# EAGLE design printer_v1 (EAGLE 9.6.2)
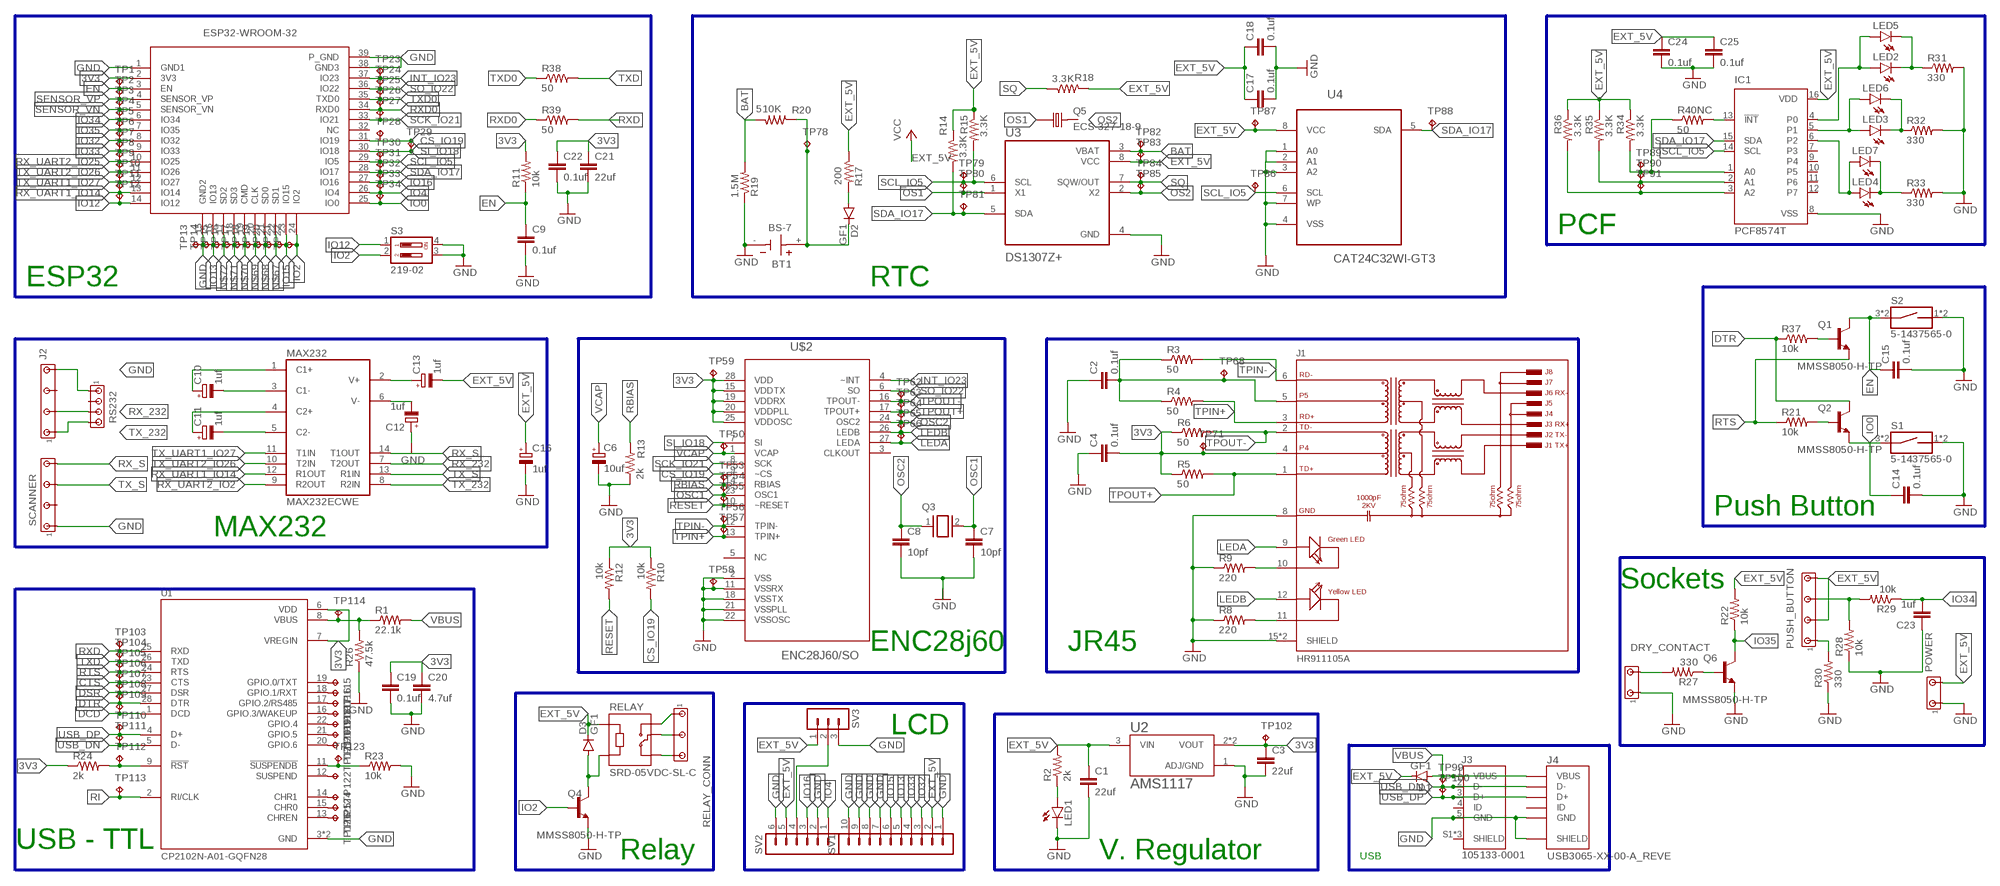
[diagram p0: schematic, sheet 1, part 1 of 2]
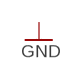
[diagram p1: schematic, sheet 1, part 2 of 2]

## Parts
BT1  BS-7  [BAT_BS-7]
C1  22uf  C-EUC1206  [C1206]
C2  0.1uf  C-EUC1206  [C1206]
C3  22uf  C-EUC1206  [C1206]
C4  0.1uf  C-EUC1206  [C1206]
C6  10uf  CPOL-EU153CLV-0405  [153CLV-0405]
C7  10pf  C-EUC1206  [C1206]
C8  10pf  C-EUC1206  [C1206]
C9  0.1uf  C-EUC1206  [C1206]
C10  1uf  CPOL-EU153CLV-0405  [153CLV-0405]
C11  1uf  CPOL-EU153CLV-0405  [153CLV-0405]
C12  1uf  CPOL-EU153CLV-0405  [153CLV-0405]
C13  1uf  CPOL-EU153CLV-0405  [153CLV-0405]
C14  0.1uf  C-EUC1206  [C1206]
C15  0.1uf  C-EUC1206  [C1206]
C16  1uf  CPOL-EU153CLV-0405  [153CLV-0405]
C17  0.1uf  C-EUC1206  [C1206]
C18  0.1uf  C-EUC1206  [C1206]
C19  0.1uf  C-EUC1206  [C1206]
C20  4.7uf  C-EUC1206  [C1206]
C21  22uf  C-EUC1206  [C1206]
C22  0.1uf  C-EUC1206  [C1206]
C23  1uf  C-EUC1206  [C1206]
C24  0.1uf  C-EUC1206  [C1206]
C25  0.1uf  C-EUC1206  [C1206]
D1  GF1  [SMA-DO214AC]
D2  GF1  [SMA-DO214AC]
D3  GF1  [SMA-DO214AC]
DRY_CONTACT  MTA03-100_MYV  [10X03MTA_MYV]
IC1  PCF8574T  [SO16W]
J1  HR911105A  [HANRUN_HR911105A]
J2  MTA07-100_MYV  [10X07MTA_MYV]
J3  105133-0001  [MOLEX_105133-0001]
J4  USB3065-XX-00-A_REVE  [GCT_USB3065-XX-00-A_REVE]
LED1  LEDSML0603  [SML0603]
LED2  LEDSML0603  [SML0603]
LED3  LEDSML0603  [SML0603]
LED4  LEDSML0603  [SML0603]
LED5  LED5MM  [LED5MM]
LED6  LED5MM  [LED5MM]
LED7  LED5MM  [LED5MM]
MAX232  MAX232ECWE  [SO16L]
POWER  MTA03-100_MYV  [10X03MTA_MYV]
PUSH_BUTTON  MTA07-100_MYV  [10X07MTA_MYV]
Q1  MMSS8050-H-TP  [TRANS_MMSS8050-H-TP]
Q2  MMSS8050-H-TP  [TRANS_MMSS8050-H-TP]
Q3  XTAL/S  [QS]
Q4  MMSS8050-H-TP  [TRANS_MMSS8050-H-TP]
Q5  ECS-327-18-9  [XTAL_ECS-160-18-9X]
Q6  MMSS8050-H-TP  [TRANS_MMSS8050-H-TP]
R1  22.1k  R-US_R1206  [R1206]
R2  2k  R-US_R1206  [R1206]
R3  50  R-US_R1206  [R1206]
R4  50  R-US_R1206  [R1206]
R5  50  R-US_R1206  [R1206]
R6  50  R-US_R1206  [R1206]
R8  220  R-US_R1206  [R1206]
R9  220  R-US_R1206  [R1206]
R10  10k  R-US_R0805  [R0805]
R11  10k  R-US_R0805  [R0805]
R12  10k  R-US_R0805  [R0805]
R13  2k  R-US_R1206  [R1206]
R14  3.3K  R-US_R1206  [R1206]
R15  3.3K  R-US_R1206  [R1206]
R17  200  R-US_R1206  [R1206]
R18  3.3K  R-US_R1206  [R1206]
R19  1.5M  R-US_R1206  [R1206]
R20  510K  R-US_R1206  [R1206]
R21  10k  R-US_R0805  [R0805]
R22  10k  R-US_R0805  [R0805]
R23  10k  R-US_R0805  [R0805]
R24  2k  R-US_R1206  [R1206]
R26  47.5k  R-US_R1206  [R1206]
R27  330  R-US_R0402  [R0402]
R28  10k  R-US_R0805  [R0805]
R29  10k  R-US_R0805  [R0805]
R30  330  R-US_R1206  [R1206]
R31  330  R-US_R1206  [R1206]
R32  330  R-US_R1206  [R1206]
R33  330  R-US_R1206  [R1206]
R34  3.3K  R-US_R1206  [R1206]
R35  3.3K  R-US_R1206  [R1206]
R36  3.3K  R-US_R1206  [R1206]
R37  10k  R-US_R0805  [R0805]
R38  50  R-US_R0402  [R0402]
R39  50  R-US_R0402  [R0402]
R40NC  50  R-US_R0402  [R0402]
RELAY  SRD-05VDC-SL-C  [RELAY_SRD-05VDC-SL-C]
RELAY_CONN  MTA05-156_MYVSPACE1  [10X05MTA_MYV]
RS232  MTA04-100  [10X04MTA]
S1  5-1437565-0  [SW_5-1437565-0]
S2  5-1437565-0  [SW_5-1437565-0]
S3  219-02  [CTS-219-02]
SCANNER  MTA07-100_MYV  [10X07MTA_MYV]
SV1  MA10-1  [MA10-1]
SV2  MA06-1  [MA06-1]
SV3  MA03-1  [MA03-1]
TP1  TPTP06R  [TP06R]
TP2  TPTP06R  [TP06R]
TP3  TPTP06R  [TP06R]
TP4  TPTP06R  [TP06R]
TP5  TPTP06R  [TP06R]
TP6  TPTP06R  [TP06R]
TP7  TPTP06R  [TP06R]
TP8  TPTP06R  [TP06R]
TP9  TPTP06R  [TP06R]
TP10  TPTP06R  [TP06R]
TP11  TPTP06R  [TP06R]
TP12  TPTP06R  [TP06R]
TP13  TPTP06R  [TP06R]
TP14  TPTP06R  [TP06R]
TP15  TPTP06R  [TP06R]
TP16  TPTP06R  [TP06R]
TP17  TPTP06R  [TP06R]
TP18  TPTP06R  [TP06R]
TP19  TPTP06R  [TP06R]
TP20  TPTP06R  [TP06R]
TP21  TPTP06R  [TP06R]
TP22  TPTP06R  [TP06R]
TP23  TPTP06R  [TP06R]
TP24  TPTP06R  [TP06R]
TP25  TPTP06R  [TP06R]
TP26  TPTP06R  [TP06R]
TP27  TPTP06R  [TP06R]
TP28  TPTP06R  [TP06R]
TP29  TPTP06R  [TP06R]
TP30  TPTP06R  [TP06R]
TP31  TPTP06R  [TP06R]
TP32  TPTP06R  [TP06R]
TP33  TPTP06R  [TP06R]
TP34  TPTP06R  [TP06R]
TP50  TPTP06R  [TP06R]
TP53  TPTP06R  [TP06R]
TP54  TPTP06R  [TP06R]
TP55  TPTP06R  [TP06R]
TP56  TPTP06R  [TP06R]
TP57  TPTP06R  [TP06R]
TP58  TPTP06R  [TP06R]
TP59  TPTP06R  [TP06R]
TP62  TPTP06R  [TP06R]
TP63  TPTP06R  [TP06R]
TP64  TPTP06R  [TP06R]
TP65  TPTP06R  [TP06R]
TP66  TPTP06R  [TP06R]
TP68  TPTP06R  [TP06R]
TP71  TPTP06R  [TP06R]
TP78  TPTP06R  [TP06R]
TP79  TPTP06R  [TP06R]
TP80  TPTP06R  [TP06R]
TP81  TPTP06R  [TP06R]
TP82  TPTP06R  [TP06R]
TP83  TPTP06R  [TP06R]
TP84  TPTP06R  [TP06R]
TP85  TPTP06R  [TP06R]
TP86  TPTP06R  [TP06R]
TP87  TPTP06R  [TP06R]
TP88  TPTP06R  [TP06R]
TP89  TPTP06R  [TP06R]
TP90  TPTP06R  [TP06R]
TP91  TPTP06R  [TP06R]
TP99  TPTP06R  [TP06R]
TP100  TPTP06R  [TP06R]
TP102  TPTP06R  [TP06R]
TP103  TPTP06R  [TP06R]
TP104  TPTP06R  [TP06R]
TP105  TPTP06R  [TP06R]
TP106  TPTP06R  [TP06R]
TP107  TPTP06R  [TP06R]
TP108  TPTP06R  [TP06R]
TP109  TPTP06R  [TP06R]
TP110  TPTP06R  [TP06R]
TP111  TPTP06R  [TP06R]
TP112  TPTP06R  [TP06R]
TP113  TPTP06R  [TP06R]
TP114  TPTP06R  [TP06R]
TP115  TPTP06R  [TP06R]
TP116  TPTP06R  [TP06R]
TP117  TPTP06R  [TP06R]
TP118  TPTP06R  [TP06R]
TP119  TPTP06R  [TP06R]
TP120  TPTP06R  [TP06R]
TP121  TPTP06R  [TP06R]
TP122  TPTP06R  [TP06R]
TP123  TPTP06R  [TP06R]
TP124  TPTP06R  [TP06R]
TP125  TPTP06R  [TP06R]
TP126  TPTP06R  [TP06R]
U1  CP2102N-A01-GQFN28  [QFN50P500X500X80-29N]
U2  AMS1117  [SOT229P700X180-4N]
U3  DS1307Z+  [SOIC127P600X175-8N]
U4  CAT24C32WI-GT3  [SOIC127P600X175-8N]
U$2  ENC28J60/SO  [SOIC127P1034X264-28N]
U$3  ESP32-WROOM-32  [ESP32-WROOM-32]

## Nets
3V3: C3.1 C4.2 C19.1 C20.1 C21.1 C22.1 J1.4 R5.1 R6.1 R10.1 R11.2 R12.1 R24.1 TP59.TP TP71.TP TP102.TP U1.6(VDD) U1.7(VREGIN) U2.2(VOUT) U2.4(VOUT) U$2.15(VDDTX) U$2.19(VDDRX) U$2.20(VDDPLL) U$2.25(VDDOSC) U$2.28(VDD) U$3.2(3V3)
BAT: R19.2 R20.2 TP82.TP U3.3(VBAT)
CS_IO19: R10.2 TP28.TP U$2.9(~CS) U$3.31(IO19)
CTS: TP106.TP U1.23(CTS)
DCD: TP109.TP U1.1(DCD)
DSR: TP107.TP U1.27(DSR)
DTR: Q2.3(C) R37.1 TP108.TP U1.28(DTR)
EN: C9.1 C15.1 Q1.3(C) R11.1 S2.3 S2.4 TP1.TP U$3.3(EN)
EXT_5V: C1.1 C13.- C16.+ C17.1 C18.1 C24.1 C25.1 D1.K(C) D3.K(C) IC1.16(VDD) POWER.3 PUSH_BUTTON.3 PUSH_BUTTON.7 R2.2 R14.1 R15.1 R17.1 R18.2 R22.2 R34.1 R35.1 R36.1 RELAY.A1 SV1.2 SV2.5 SV3.1 TP83.TP TP87.TP U2.3(VIN) U3.8(VCC) U4.8(VCC) ; supply symbol labelled VCC
GND: BT1.- C1.2 C2.1 C3.2 C4.1 C6.- C7.2 C8.2 C9.2 C12.+ C14.2 C15.2 C16.- C17.2 C18.2 C19.2 C20.2 C21.2 C22.2 C23.1 C24.2 C25.2 DRY_CONTACT.1 IC1.8(VSS) J1.8(GND) J1.15(SHIELD) J1.16(SHIELD) J2.7 J3.5(GND) J4.5(GND) J4.6(SHIELD) J4.7(SHIELD) J4.8(SHIELD) J4.9(SHIELD) LED1.C POWER.1 Q4.2(E) Q6.2(E) R8.1 R9.1 R13.1 R19.1 R23.2 R26.1 R28.1 R30.1 R31.2 R32.2 R33.2 RS232.1 S1.1 S1.2 S2.1 S2.2 S3.3 S3.4 SCANNER.1 SV1.1 SV1.7 SV1.8 SV1.9 SV1.10 SV2.2 SV2.6 SV3.3 TP13.TP TP58.TP U1.3(GND) U1.29(GND) U2.1(ADJ/GND) U3.4(GND) U4.1(A0) U4.2(A1) U4.3(A2) U4.4(VSS) U4.7(WP) U$2.2(VSS) U$2.11(VSSRX) U$2.18(VSSTX) U$2.21(VSSPLL) U$2.22(VSSOSC) U$3.1(GND1) U$3.15(GND2) U$3.38(GND3) U$3.39(P_GND)
INT_IO23: TP23.TP U$2.4(~INT) U$3.37(IO23)
IO0: C14.1 Q2.2(E) S1.3 S1.4 TP34.TP U$3.25(IO0)
IO2: Q4.1(B) S3.2 TP22.TP U$3.24(IO2)
IO4: SV2.1 TP33.TP U$3.26(IO4)
IO12: S3.1 TP12.TP U$3.14(IO12)
IO13: SV1.5 TP14.TP U$3.16(IO13)
IO15: SV1.6 TP21.TP U$3.23(IO15)
IO16: SV2.3 TP32.TP U$3.27(IO16)
IO32: SV1.3 TP6.TP U$3.8(IO32)
IO33: SV1.4 TP7.TP U$3.9(IO33)
IO34: C23.2 R29.1 TP4.TP U$3.6(IO34)
IO35: Q6.3(C) R22.1 TP5.TP U$3.7(IO35)
LEDA: J1.9(GA) TP66.TP U$2.27(LEDA)
LEDB: J1.12(YA) TP65.TP U$2.26(LEDB)
N$1: LED1.A R2.1
N$2: Q1.1(B) R37.2
N$3: Q2.1(B) R21.2
N$4: R1.1 R26.2 TP114.TP U1.8(VBUS)
N$5: SV2.4 SV3.2
N$6: R23.1 TP123.TP U1.11(!SUSPENDB)
N$7: J1.11(YC) R8.2
N$8: C2.2 J1.5 R3.1 R4.1 TP68.TP
N$9: J1.10(GC) R9.2
N$10: TP115.TP U1.19(GPIO.0/TXT)
N$11: TP116.TP U1.18(GPIO.1/RXT)
N$12: C10.+ MAX232.1(C1+)
N$13: TP117.TP U1.17(GPIO.2/RS485)
N$14: C10.- MAX232.3(C1-)
N$15: C11.- MAX232.5(C2-)
N$16: R24.2 TP112.TP U1.9(!RST)
N$17: TP118.TP U1.16(GPIO.3/WAKEUP)
N$18: C11.+ MAX232.4(C2+)
N$19: C12.- MAX232.6(V-)
N$20: C13.+ MAX232.2(V+)
N$21: RELAY.NC RELAY_CONN.5
N$22: RELAY.COM RELAY_CONN.3
N$23: LED2.C LED5.K(C) R31.1
N$24: IC1.13(!INT) R40NC.2
N$25: TP119.TP U1.22(GPIO.4)
N$26: RELAY.NO RELAY_CONN.1
N$27: D3.A Q4.3(C) RELAY.A2
N$28: D2.A R17.2
N$29: BT1.+ D2.K(C) R20.1 TP78.TP
N$30: TP120.TP U1.21(GPIO.5)
N$31: TP121.TP U1.20(GPIO.6)
N$32: Q6.1(B) R27.1
N$33: PUSH_BUTTON.5 R28.2 R29.2
N$34: TP122.TP U1.12(SUSPEND)
N$35: DRY_CONTACT.3 R27.2
N$36: IC1.4(P0) LED2.A LED5.A
N$37: IC1.5(P1) LED3.A LED6.A
N$38: IC1.6(P2) LED4.A LED7.A
N$39: TP124.TP U1.14(CHR1)
N$40: PUSH_BUTTON.1 R30.2
N$41: TP125.TP U1.15(CHR0)
N$42: TP126.TP U1.13(CHREN)
N$45: IC1.1(A0) R34.2 R40NC.1 TP89.TP
N$46: IC1.2(A1) R35.2 TP90.TP
N$47: IC1.3(A2) R36.2 TP91.TP
N$48: LED3.C LED6.K(C) R32.1
N$49: LED4.C LED7.K(C) R33.1
N$67: TP20.TP U$3.22(SD1)
N$68: TP19.TP U$3.21(SD0)
N$69: TP18.TP U$3.20(CLK)
N$70: TP17.TP U$3.19(CMD)
N$71: TP16.TP U$3.18(SD3)
N$72: TP15.TP U$3.17(SD2)
OS1: Q5.1 TP80.TP U3.1(X1)
OS2: Q5.2 TP85.TP U3.2(X2)
OSC1: C7.1 Q3.2 TP54.TP U$2.23(OSC1)
OSC2: C8.1 Q3.1 TP64.TP U$2.24(OSC2)
RBIAS: R13.2 TP53.TP U$2.14(RBIAS)
RESET: R12.2 TP55.TP U$2.10(~RESET)
RI: TP113.TP U1.2(RI/CLK)
RTS: Q1.2(E) R21.1 TP105.TP U1.24(RTS)
RX_232: J2.3 MAX232.7(T2OUT) RS232.3
RX_S: MAX232.14(T1OUT) SCANNER.7
RX_UART1_IO14: MAX232.12(R1OUT) TP11.TP U$3.13(IO14)
RX_UART2_IO2: MAX232.9(R2OUT)
RX_UART2_IO25: TP8.TP U$3.10(IO25)
RXD: R39.2 TP103.TP U1.25(RXD)
RXD0: R39.1 TP26.TP U$3.34(RXD0)
SCK_IO21: TP27.TP U$2.8(SCK) U$3.33(IO21)
SCL_IO5: IC1.14(SCL) R15.2 TP30.TP TP79.TP TP86.TP U3.6(SCL) U4.6(SCL) U$3.29(IO5)
SDA_IO17: IC1.15(SDA) R14.2 TP31.TP TP81.TP TP88.TP U3.5(SDA) U4.5(SDA) U$3.28(IO17)
SENSOR_VN: TP3.TP U$3.5(SENSOR_VN)
SENSOR_VP: TP2.TP U$3.4(SENSOR_VP)
SI_IO18: TP29.TP U$2.7(SI) U$3.30(IO18)
SO_IO22: TP24.TP U$2.6(SO) U$3.36(IO22)
SQ: R18.1 TP84.TP U3.7(SQW/OUT)
TPIN+: J1.3(RD+) R4.2 TP57.TP U$2.13(TPIN+)
TPIN-: J1.6(RD-) R3.2 TP56.TP U$2.12(TPIN-)
TPOUT+: J1.1(TD+) R5.2 TP63.TP U$2.17(TPOUT+)
TPOUT-: J1.2(TD-) R6.2 TP62.TP U$2.16(TPOUT-)
TX_232: J2.1 MAX232.8(R2IN) RS232.4
TX_S: MAX232.13(R1IN) SCANNER.5
TX_UART1_IO27: MAX232.11(T1IN) TP10.TP U$3.12(IO27)
TX_UART2_IO26: MAX232.10(T2IN) TP9.TP U$3.11(IO26)
TXD: R38.2 TP104.TP U1.26(TXD)
TXD0: R38.1 TP25.TP U$3.35(TXD0)
USB_DN: J3.2(D-) J4.2(D-) TP99.TP TP111.TP U1.5(D-)
USB_DP: J3.3(D+) J4.3(D+) TP100.TP TP110.TP U1.4(D+)
VBUS: D1.A J3.1(VBUS) J4.1(VBUS) R1.2
VCAP: C6.+ TP50.TP U$2.1(VCAP)
Unconnected: IC1.7(P3) IC1.9(P4) IC1.10(P5) IC1.11(P6) IC1.12(P7) J2.5 J3.4(ID) J3.S1(SHIELD) J3.S2(SHIELD) J3.S3(SHIELD) J4.4(ID) RS232.2 SCANNER.3 U$2.3(CLKOUT) U$2.5(NC) U$3.32(NC)

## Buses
B$1
B$2
BAT,EXT_5V,GND,N$28,N$29
B$3
B$4
B$5
B$6
B$7
GND,EXT_5V_PIN
B$8
VBUS,GND,USB_DN,N$6,3V3,RI,RTS,RXD,TXD,CTS,DSR,N$4,DTR,DCD,USB_DP,N$16
B$9
B$10

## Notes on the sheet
- PCF
- ESP32 | RTC
- Push Button
- MAX232
- Sockets
- ENC28j60 | JR45
- LCD
- USB - TTL
- Relay | V. Regulator | USB

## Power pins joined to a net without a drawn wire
EXT_5V: MAX232.16(VCC)
GND: MAX232.15(GND)

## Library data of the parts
BT1 = BS-7:BS-7: BATTERY HOLDER COIN 20MM PC PIN; AVAILABILITY: Unavailable; DESCRIPTION: BATTERY HOLDER COIN 20MM PC PIN; MF: MPD _Memory; MP: BS-7; PACKAGE: None; PRICE: None
C1-C4 C7-C9 C14 C15 C17-C25 = rcl:C-EU: CAPACITOR, European symbol; SPICEPREFIX: C
C6 C10-C13 C16 = rcl:CPOL-EU: POLARIZED CAPACITOR, European symbol; SPICEPREFIX: C
D1-D3 = diode:GF1: DIODE
DRY_CONTACT POWER = con-amp_edit:MTA03-100_MYV: AMP connector
IC1 = micro-philips:PCF8574: I2C-Bus Remote 8-bit I/O expander http://www.semiconductors.philips.com/acrobat_download/datasheets/PCF8574_4.pdf; MPN: PCF8574T/3,512; OC_FARNELL: 1201255; OC_NEWARK: 70R6870
J1 = HR911105A:HR911105A: DIP RJ45 Connector;; AVAILABILITY: Unavailable; DESCRIPTION: HR911105A Ethernet Interface Arduino Platform Evaluation Expansion Board; MF: DFRobot; MP: HR911105A; PACKAGE: None; PRICE: None
J2 PUSH_BUTTON SCANNER = con-amp_edit:MTA07-100_MYV: AMP connector
J3 = 105133-0001:105133-0001: Conn Micro USB Type B RCP 5 POS 0.65mm Solder RA SMD 5 Terminal 1 Port Embossed T/R; AVAILABILITY: Unavailable; DESCRIPTION: USB - micro B USB 2.0 Receptacle Connector 5 Position Surface Mount; MF: Molex; MP: 105133-0001; PACKAGE: None; PRICE: None
J4 = USB3065-XX-00-A_REVE:USB3065-XX-00-A_REVE: Micro USB Receptacle, Type B, 5 Pin, SMT, Horizontal, Bottom Mount (Standart), Optional Plastic Locating Peg; AVAILABILITY: Unavailable; DESCRIPTION: USB3065 Series 5 Pin, SMT, Horizontal, Bottom Mount, Micro USB Receptacle; MF: Global Connector Technology; MP: USB3065-30-00-A; PACKAGE: None; PRICE: None
LED1-LED4 = led:LED: LED
LED5-LED7 = led_MYVV:LED: LED
MAX232 = maxim:MAX232ECWE: RS232 TRANSCEIVER; MF: MAXIM; MPN: MAX232ECWE+; OC_FARNELL: 9724435; OC_NEWARK: 67K4440
Q1 Q2 Q4 Q6 = MMSS8050-H-TP:MMSS8050-H-TP: MMSS8050-H Series 25 V 1.5 A NPN Silicon Plastic-Encapsulate Transistor-SOT-23; AVAILABILITY: Unavailable; DESCRIPTION: Bipolar _BJT_ Transistor NPN 25V 1.5A 100MHz 625mW Surface Mount SOT-23; MF: Micro Commercial; MP: MMSS8050-H-TP; PACKAGE: SOT-23 Micro Commercial; PRICE: None
Q3 = special:XTAL/S: CRYSTAL
Q5 = ECS-327-18-9:ECS-327-18-9: Crystal Cylindrical Can, Radial; AVAILABILITY: Unavailable; DESCRIPTION: 32.768MHz ±50ppm Crystal 18pF 100 Ohms Cylindrical Can, Radial; MF: ECS International; MP: ECS-327-18-9; PACKAGE: Cylindrical Can Radial ECS International; PRICE: None
R1-R6 R8-R15 R17-R24 R26-R39 R40NC = rcl:R-US_: RESISTOR, American symbol; SPICEPREFIX: R
RELAY = SRD-05VDC-SL-C:SRD-05VDC-SL-C: 5V Trigger Relay Module For Arduino And Raspberry Pi 5V Trigger Relay Module For Arduino And Raspberry Pi; AVAILABILITY: Unavailable; DESCRIPTION: 5V Trigger Relay Module For Arduino And Raspberry Pi 5V Trigger Relay Module For Arduino And Raspberry Pi; MF: Songle Relay; MP: SRD-05VDC-SL-C; PACKAGE: None; PRICE: None
RELAY_CONN = con-amp_edit:MTA05-156_MYV: AMP connector
RS232 = con-amp:MTA04-100: AMP connector
S1 S2 = 5-1437565-0:5-1437565-0: Switch Tactile OFF (ON) Round Button Gull Wing 0.05A 12VDC 1.57N SMD T/R; AVAILABILITY: Unavailable; COMMENT: 5-1437565-0; DESCRIPTION: Switch Push Button N.O. SPST Round Button 0.05A 12VDC 1VA Alternate Contact Gull Wing SMD T/R; MF: TE Connectivity; MP: FSM6JSMATR; PACKAGE: None; PRICE: None; TE_PURCHASE_URL: https://www.te.com/usa-en/product-5-1437565-0.html?te_bu=Cor&te_type=disp&te_campaign=seda_glo_cor-seda-global-disp-prtnr-fy19-seda-model-bom-cta_sma-317_1&elqCampaignId=32493
S3 = switch-dil:219-02*: Surface Mount DIP Switch Series 219 SMT CTS Electronic Components Sourc: www.ctscorp.com; OC_FARNELL: unknown; OC_NEWARK: unknown
SV1 = con-lstb:MA10-1: PIN HEADER; OC_FARNELL: unknown; OC_NEWARK: unknown
SV2 = con-lstb:MA06-1: PIN HEADER; OC_FARNELL: unknown; OC_NEWARK: unknown
SV3 = con-lstb:MA03-1: PIN HEADER; OC_FARNELL: unknown; OC_NEWARK: unknown
TP1-TP34 TP50 TP53-TP59 TP62-TP66 TP68 TP71 TP78-TP91 TP99 TP100 TP102-TP126 = testpad:TP: Test pad
U1 = CP2102N-A01-GQFN28:CP2102N-A01-GQFN28: Ic Bridge Usb To Uart 28qfn; DESCRIPTION: USB Bridge, USB to UART USB 2.0 UART Interface 28-QFN _5x5_; DIGI-KEY_PART_NUMBER: 336-3694-ND; DIGI-KEY_PURCHASE_URL: https://www.digikey.com/product-detail/en/silicon-labs/CP2102N-A01-GQFN28/336-3694-ND/6012519?utm_source=snapeda&utm_medium=aggregator&utm_campaign=symbol; MF: Silicon Labs; MP: CP2102N-A01-GQFN28; PACKAGE: QFN-28 Silicon Labs
U2 = AMS1117:AMS1117: Sot223/Pkg 1-Amp 5-Volt Low Drop Out Voltage Regulatator; AVAILABILITY: Unavailable; DESCRIPTION: UNO PLUS Arduino R3 Shield, Xbee Arduino IDE Wheeled Robotics Kit; MF: Seeed Technology; MP: AMS1117; PACKAGE: SOT-223 Seeed Technology; PRICE: None
U3 = DS1307Z_:DS1307Z+; AVAILABILITY: Unavailable; DESCRIPTION: Real Time Clock _RTC_ IC Clock/Calendar 56B I²C, 2-Wire Serial 8-SOIC _0.154, 3.90mm Width_; MF: Maxim Integrated; MP: DS1307Z; PACKAGE: SO-8 Maxim Integrated; PRICE: None
U4 = CAT24C32WI-GT3:CAT24C32WI-GT3: 32-Kb I2C CMOS Serial EEPROM; AVAILABILITY: Unavailable; DESCRIPTION: EEPROM Memory IC 32Kb _4K x 8_ I²C 1MHz 400ns 8-SOIC; MF: ON; MP: CAT24C32WI-GT3; PACKAGE: SOIC-8 ON; PRICE: None
U$2 = ENC28J60_SO:ENC28J60/SO: Stand-Alone Ethernet Controller;; AVAILABILITY: Unavailable; DESCRIPTION: Ethernet Controller 10 Base-T PHY SPI Interface 28-SSOP; MF: Microchip; MP: ENC28J60/SS; PACKAGE: SSOP-28 Microchip; PRICE: None
U$3 = ESP32-WROOM-32:ESP32-WROOM-32: ESP32-WROOM-32 Module; AVAILABILITY: Unavailable; DESCRIPTION: Bluetooth, WiFi Transceiver Module 2.4GHz ~ 2.5GHz Surface Mount; MF: Espressif Systems; MP: ESP32-WROOM-32; PACKAGE: Module Espressif Systems; PRICE: None

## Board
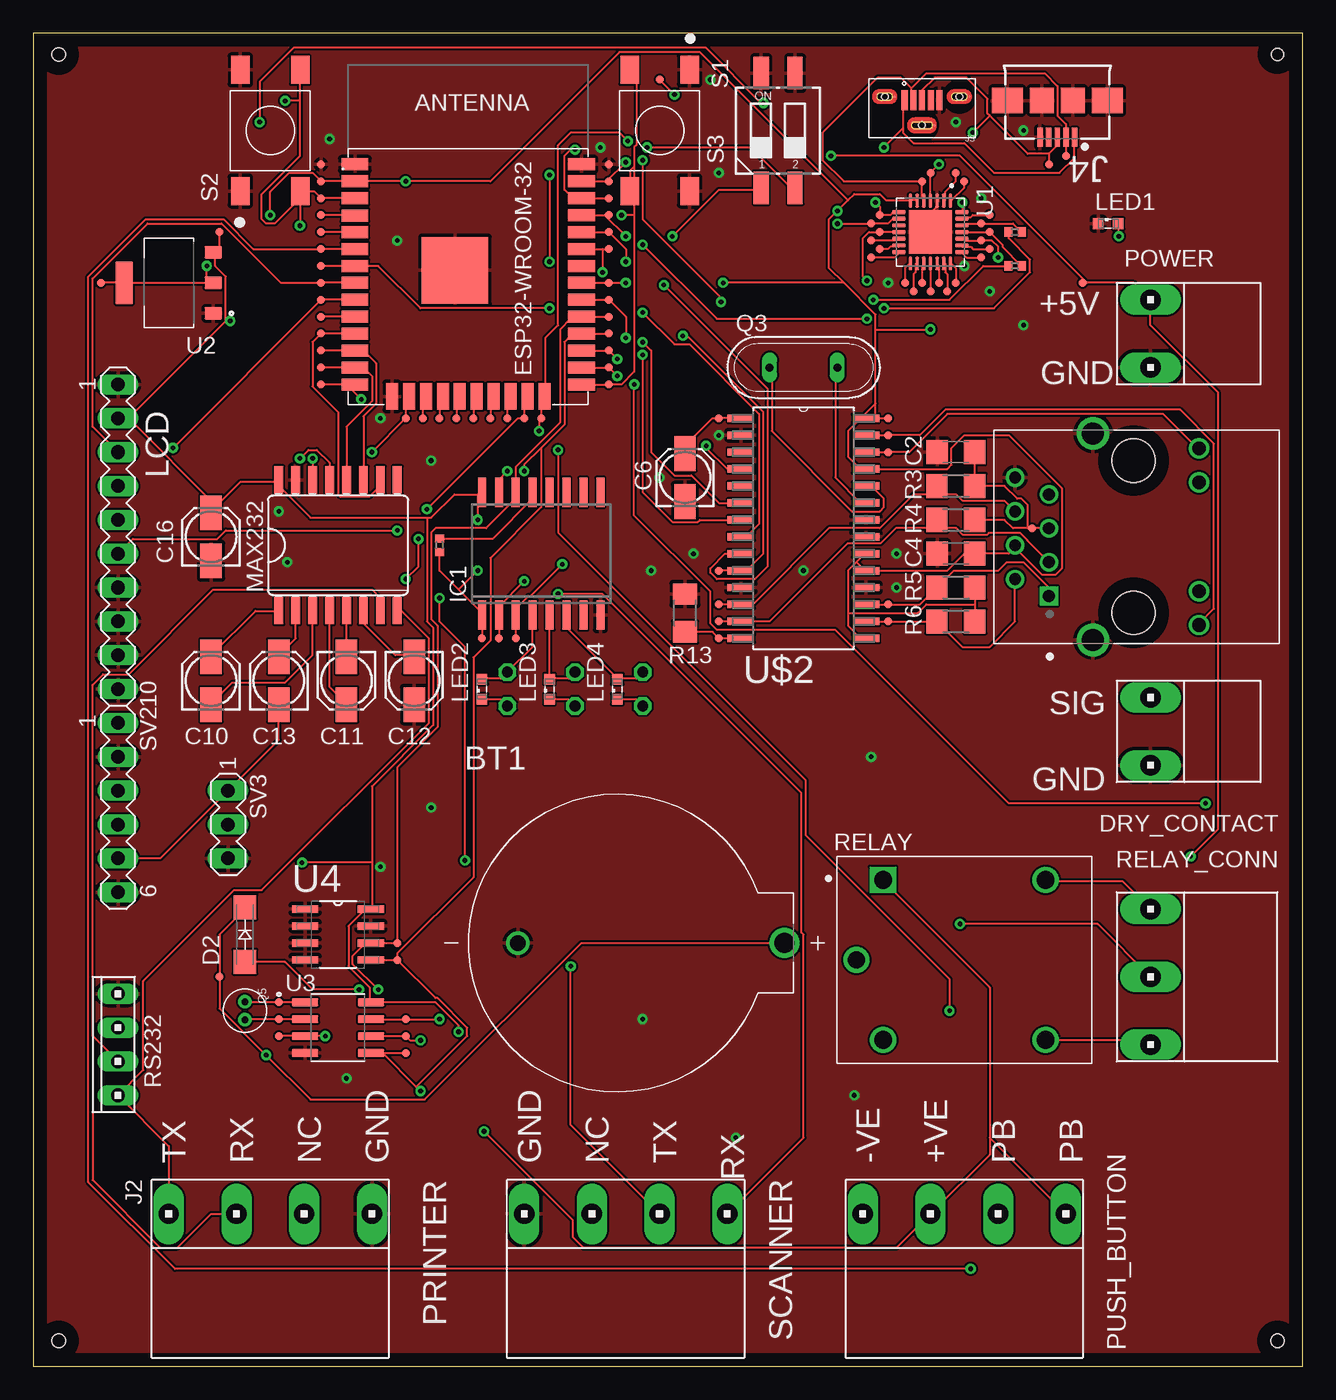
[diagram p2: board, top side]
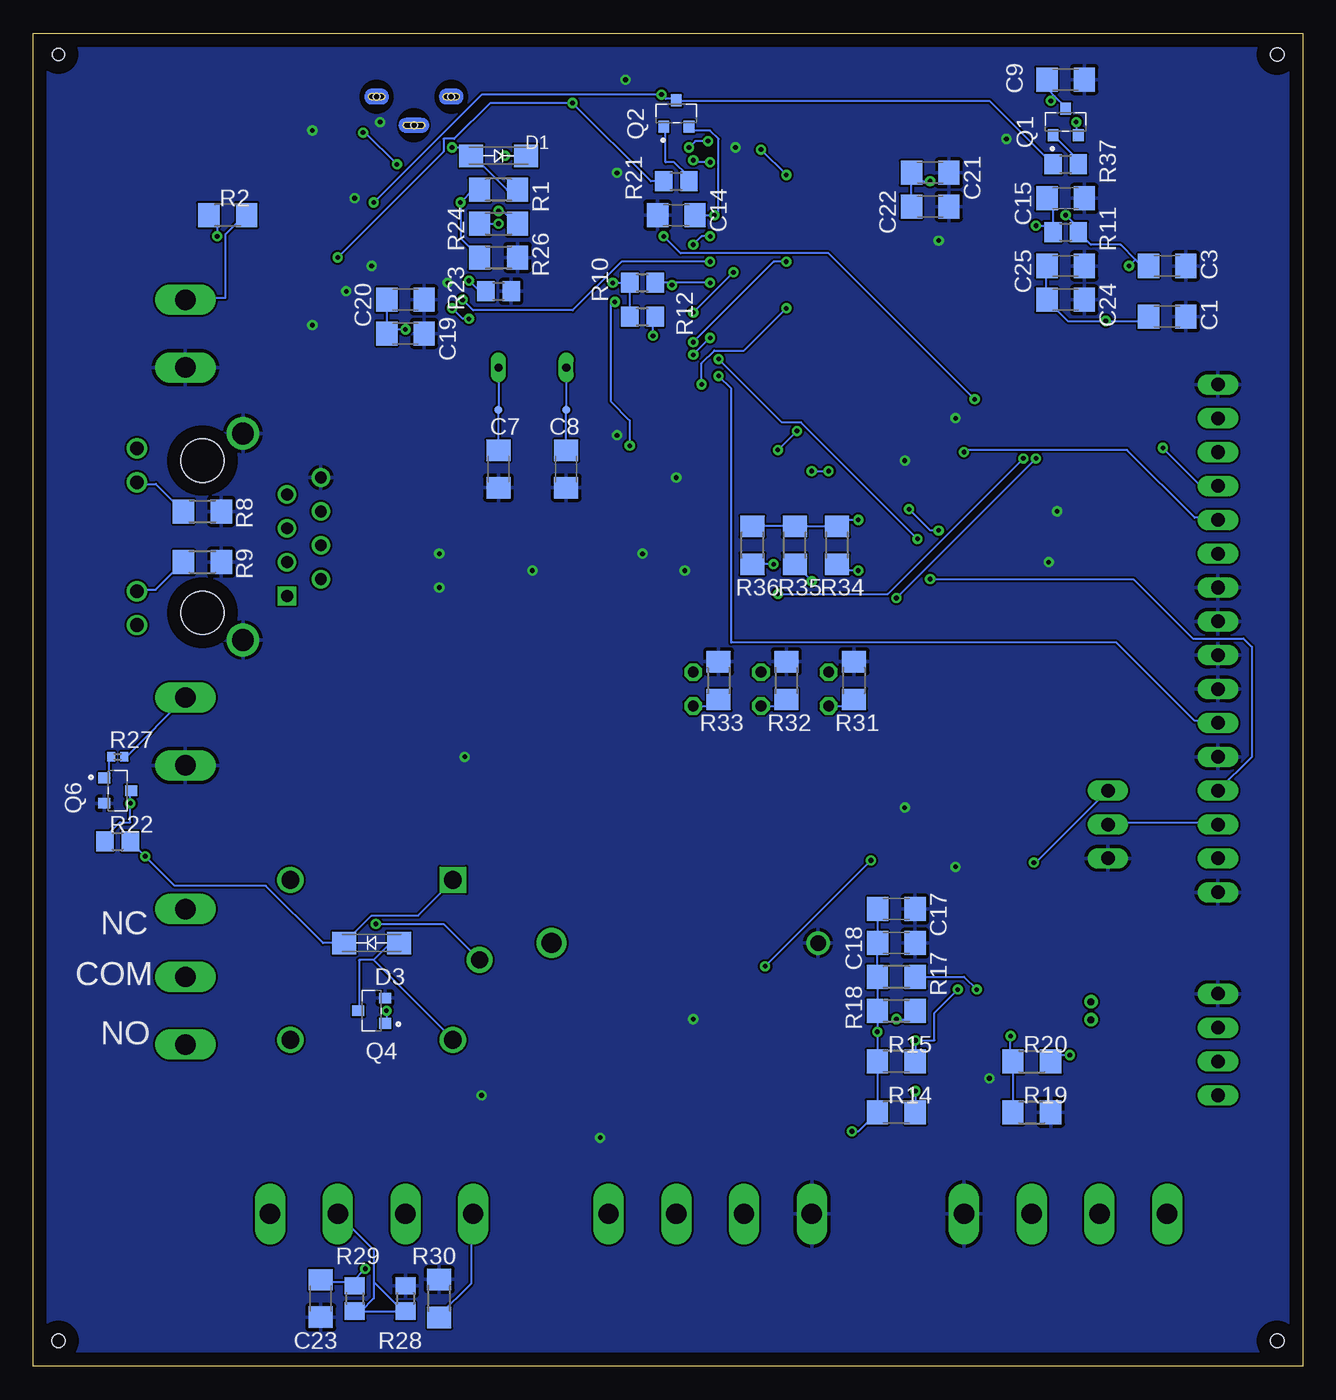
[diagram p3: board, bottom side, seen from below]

Size 95.23 x 100 mm. Coordinates in mm from the lower left corner, seen from the top.
Outline: 0,0 95.23,0 95.23,100 0,100 0,0
Copper layers (1*16): Top 0.035mm / dielectric 1.5mm / Bottom 0.035mm
Design rules "default": minimum track width 6mil, minimum drill 0.35mm, track to track 6mil, track to pad 6mil, pad to pad 6mil, via to via 6mil, smd to smd 6mil, copper to edge 40mil, drill to drill 6mil, minimum pad ring 10mil, minimum via ring 8mil, stop-mask expansion 4mil, vias tented up to drill 0mil, thermal gap 10mil
Holes 1 mm at 1.91,1.91 93.34,1.91 1.91,98.42
Holes 0.9 mm at 93.34,98.42

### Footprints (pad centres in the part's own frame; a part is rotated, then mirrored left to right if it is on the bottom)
BAT_BS-7 = drill 1.5: + 10,0 | drill 1.17: - -10,0
C1206 = smd 1.6 x 1.8: 1 -1.4,0; 2 1.4,0
153CLV-0405 = smd 2.6 x 1.6: + 1.8,0; - -1.8,0
SMA-DO214AC = smd 1.8 x 1.7: A -2.05,0; K 2.05,0
10X03MTA_MYV = drill 1.524 long: 1 2.54,0; 3 -2.54,0
SO16W = smd 0.6 x 2.2: 1 -4.445,-4.6; 2 -3.175,-4.6; 3 -1.905,-4.6; 4 -0.635,-4.6; 5 0.635,-4.6; 6 1.905,-4.6; 7 3.175,-4.6; 8 4.445,-4.6; 9 4.445,4.6; 10 3.175,4.6; 11 1.905,4.6; 12 0.635,4.6; 13 -0.635,4.6; 14 -1.905,4.6; 15 -3.175,4.6; 16 -4.445,4.6
HANRUN_HR911105A = drill 0.89 square: 1 4.45,-6.35 | drill 0.89: 2 3.18,-8.89; 3 1.91,-6.35; 4 0.64,-8.89; 5 -0.63,-6.35; 6 -1.9,-8.89; 7 -3.17,-6.35; 8 -4.44,-8.89 | drill 1.02: 9 6.625,4.9; 10 4.085,4.9; 11 -4.085,4.9; 12 -6.625,4.9 | drill 1.63: 15 7.745,-3.05; 16 -7.745,-3.05 | hole 3.25: -5.715,0; 5.715,0
10X07MTA_MYV = drill 1.524 long: 1 7.62,0; 3 2.54,0; 5 -2.54,0; 7 -7.62,0
MOLEX_105133-0001 = smd 0.45 x 1.5: 1 -1.3,-0.25; 2 -0.65,-0.25; 3 0,-0.25; 4 0.65,-0.25; 5 1.3,-0.25 | smd 0.1 x 0.1: S1 -2.05,0; S2 3.55,0; S3 0.95,-2.15 | hole 0.5: -2.8,0; 2.8,0; 0,-2.15
GCT_USB3065-XX-00-A_REVE = smd 0.4 x 1.4: 1 -1.3,0.5; 2 -0.65,0.5; 3 0,0.5; 4 0.65,0.5; 5 1.3,0.5 | smd 1.8 x 1.9: 6 1.15,-2.25; 7 -1.15,-2.25 | smd 2.3 x 1.9: 8 3.75,-2.25; 9 -3.75,-2.25
SML0603 = smd 0.8 x 0.8: A 0.75,0; C -0.75,0
LED5MM = drill 0.813 octagon: A -1.27,0; K 1.27,0
SO16L = smd 0.66 x 2.032: 1 -4.445,-4.902; 2 -3.175,-4.902; 3 -1.905,-4.902; 4 -0.635,-4.902; 5 0.635,-4.902; 6 1.905,-4.902; 7 3.175,-4.902; 8 4.445,-4.902; 9 4.445,4.902; 10 3.175,4.902; 11 1.905,4.902; 12 0.635,4.902; 13 -0.635,4.902; 14 -1.905,4.902; 15 -3.175,4.902; 16 -4.445,4.902
TRANS_MMSS8050-H-TP = smd 0.9 x 0.8: 1 -1,0.95; 2 -1,-0.95; 3 1,0
QS = drill 0.61 long: 1 -2.54,0; 2 2.54,0
XTAL_ECS-160-18-9X = drill 0.52 pad 0.92: 1 -0.677,0; 2 0.677,0
R1206 = smd 1.6 x 1.803: 1 -1.422,0; 2 1.422,0
R0805 = smd 1.3 x 1.5: 1 -0.95,0; 2 0.95,0
R0402 = smd 0.6 x 0.7: 1 -0.5,0; 2 0.5,0
RELAY_SRD-05VDC-SL-C = drill 1.32 square: A1 -6.1,6 | drill 1.32: A2 -6.1,-6; NC 6.1,6; NO 6.1,-6 | drill 1.29: COM -8.1,0
10X05MTA_MYV = drill 1.524 long: 1 5.08,0; 3 0,0; 5 -5.08,0
10X04MTA = drill 1.016 long: 1 3.81,0; 2 1.27,0; 3 -1.27,0; 4 -3.81,0
SW_5-1437565-0 = smd 2.1 x 1.4: 1 -4.55,2.25; 2 4.55,2.25; 3 -4.55,-2.25; 4 4.55,-2.25
CTS-219-02 = smd 1.13 x 2.44: 1 -1.27,-4.3; 2 1.27,-4.3; 3 1.27,4.3; 4 -1.27,4.3
MA10-1 = drill 1.016 long: 1 -11.43,0; 2 -8.89,0; 3 -6.35,0; 4 -3.81,0; 5 -1.27,0; 6 1.27,0; 7 3.81,0; 8 6.35,0; 9 8.89,0; 10 11.43,0
MA06-1 = drill 1.016 long: 1 -6.35,0; 2 -3.81,0; 3 -1.27,0; 4 1.27,0; 5 3.81,0; 6 6.35,0
MA03-1 = drill 1.016 long: 1 -2.54,0; 2 0,0; 3 2.54,0
TP06R = smd 0.6 x 0.6: TP 0,0
QFN50P500X500X80-29N = smd 1.01 x 0.27: 1 -2.36,1.5; 2 -2.36,1; 3 -2.36,0.5; 4 -2.36,0; 5 -2.36,-0.5; 6 -2.36,-1; 7 -2.36,-1.5; 15 2.36,-1.5; 16 2.36,-1; 17 2.36,-0.5; 18 2.36,0; 19 2.36,0.5; 20 2.36,1; 21 2.36,1.5 | smd 0.27 x 1.01: 8 -1.5,-2.36; 9 -1,-2.36; 10 -0.5,-2.36; 11 0,-2.36; 12 0.5,-2.36; 13 1,-2.36; 14 1.5,-2.36; 22 1.5,2.36; 23 1,2.36; 24 0.5,2.36; 25 0,2.36; 26 -0.5,2.36; 27 -1,2.36; 28 -1.5,2.36 | smd 3.25 x 3.25: 29 0,0
SOT229P700X180-4N = smd 1.31 x 0.93: 1 -3.345,2.29; 2 -3.345,0; 3 -3.345,-2.29 | smd 1.31 x 3.24: 4 3.345,0
SOIC127P600X175-8N = smd 1.97 x 0.59: 1 -2.475,1.905; 2 -2.475,0.635; 3 -2.475,-0.635; 4 -2.475,-1.905; 5 2.475,-1.905; 6 2.475,-0.635; 7 2.475,0.635; 8 2.475,1.905
SOIC127P600X175-8N' = smd 1.981 x 0.559: 1 -2.464,1.905; 2 -2.464,0.635; 3 -2.464,-0.635; 4 -2.464,-1.905; 5 2.464,-1.905; 6 2.464,-0.635; 7 2.464,0.635; 8 2.464,1.905
SOIC127P1034X264-28N = smd 1.981 x 0.559: 1 -4.699,8.255; 2 -4.699,6.985; 3 -4.699,5.715; 4 -4.699,4.445; 5 -4.699,3.175; 6 -4.699,1.905; 7 -4.699,0.635; 8 -4.699,-0.635; 9 -4.699,-1.905; 10 -4.699,-3.175; 11 -4.699,-4.445; 12 -4.699,-5.715; 13 -4.699,-6.985; 14 -4.699,-8.255; 15 4.699,-8.255; 16 4.699,-6.985; 17 4.699,-5.715; 18 4.699,-4.445; 19 4.699,-3.175; 20 4.699,-1.905; 21 4.699,-0.635; 22 4.699,0.635; 23 4.699,1.905; 24 4.699,3.175; 25 4.699,4.445; 26 4.699,5.715; 27 4.699,6.985; 28 4.699,8.255
ESP32-WROOM-32 = smd 2 x 0.9: 1 0,0; 2 0,-1.27; 3 -0.01,-2.54; 4 0,-3.84; 5 0,-5.08; 6 0,-6.35; 7 0,-7.62; 8 0,-8.89; 9 0,-10.16; 10 0,-11.43; 11 0,-12.7; 12 0,-13.97; 13 0,-15.24; 14 0,-16.51; 25 16.999,-16.511; 26 16.999,-15.239; 27 17.001,-13.971; 28 16.999,-12.702; 29 16.997,-11.432; 30 16.999,-10.161; 31 17.002,-8.891; 32 17,-7.622; 33 17,-6.35; 34 17,-5.08; 35 17,-3.81; 36 17,-2.54; 37 17,-1.27; 38 17,0 | smd 0.9 x 2: 15 2.785,-17.41; 16 4.055,-17.41; 17 5.325,-17.41; 18 6.595,-17.41; 19 7.865,-17.41; 20 9.135,-17.41; 21 10.405,-17.41; 22 11.675,-17.41; 23 12.945,-17.41; 24 14.215,-17.41 | smd 5 x 5: 39 7.502,-7.946

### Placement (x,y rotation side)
BT1  46.35,31.75 0 top
C1  10.16,78.74 0 bottom
C2  69.22,68.58 0 top
C3  10.16,82.55 0 bottom
C4  69.22,60.96 0 top
C6  48.9,66.67 90 top
C7  60.33,67.31 270 bottom
C8  55.24,67.31 270 bottom
C9  17.78,96.52 0 bottom
C10  13.34,51.44 90 top
C11  23.5,51.44 270 top
C12  28.57,51.44 270 top
C13  18.41,51.44 90 top
C14  46.99,86.36 180 bottom
C15  17.78,87.63 0 bottom
C16  13.34,62.23 90 top
C17  30.48,34.29 0 bottom
C18  30.48,31.75 0 bottom
C19  67.31,77.47 0 bottom
C20  67.31,80.01 0 bottom
C21  27.94,89.53 0 bottom
C22  27.94,87 0 bottom
C23  73.66,5.08 90 bottom
C24  17.78,80.01 0 bottom
C25  17.78,82.55 0 bottom
D1  60.33,90.81 0 bottom
D2  15.88,32.38 90 top
D3  69.85,31.75 180 bottom
DRY_CONTACT  83.82,47.62 270 top
IC1  38.1,60.96 0 top
J1  82.55,62.23 270 top
J2  17.78,11.43 180 top
J3  66.67,95.25 0 top
J4  76.83,92.71 180 top
LED1  80.64,85.72 0 top
LED2  33.66,50.8 90 top
LED3  38.73,50.8 90 top
LED4  43.81,50.8 90 top
LED5  35.56,50.8 270 top
LED6  40.64,50.8 270 top
LED7  45.72,50.8 270 bottom
MAX232  22.86,61.59 0 top
POWER  83.82,77.47 270 top
PUSH_BUTTON  69.85,11.43 180 top
Q1  17.78,93.34 90 bottom
Q2  46.99,93.98 90 bottom
Q3  57.78,74.93 0 top
Q4  69.85,26.67 180 bottom
Q5  15.88,26.67 270 top
Q6  88.9,43.18 0 bottom
R1  60.33,88.27 0 bottom
R2  80.64,86.36 0 bottom
R3  69.22,66.04 180 top
R4  69.22,63.5 180 top
R5  69.22,58.42 180 top
R6  69.22,55.88 180 top
R8  82.55,64.14 180 bottom
R9  82.55,60.33 180 bottom
R10  49.53,81.28 0 bottom
R11  17.78,85.09 0 bottom
R12  49.53,78.74 0 bottom
R13  48.9,56.52 270 top
R14  30.48,19.05 0 bottom
R15  30.48,22.86 0 bottom
R17  30.48,29.21 0 bottom
R18  30.48,26.67 180 bottom
R19  20.32,19.05 180 bottom
R20  20.32,22.86 180 bottom
R21  46.99,88.9 0 bottom
R22  88.9,39.37 0 bottom
R23  60.33,80.64 0 bottom
R24  60.33,85.72 180 bottom
R26  60.33,83.19 180 bottom
R27  88.9,45.72 0 bottom
R28  67.31,5.08 270 bottom
R29  71.12,5.08 270 bottom
R30  64.77,5.08 270 bottom
R31  33.66,51.44 90 bottom
R32  38.73,51.44 90 bottom
R33  43.81,51.44 90 bottom
R34  34.92,61.59 270 bottom
R35  38.1,61.59 270 bottom
R36  41.27,61.59 270 bottom
R37  17.78,90.17 0 bottom
R38  73.66,85.09 0 top
R39  73.66,82.55 0 top
R40NC  30.48,61.59 90 top
RELAY  69.85,30.48 0 top
RELAY_CONN  83.82,29.21 270 top
RS232  6.35,24.13 90 top
S1  46.99,92.71 270 top
S2  17.78,92.71 90 top
S3  55.88,92.71 0 top
SCANNER  44.45,11.43 180 top
SV1  6.35,62.23 270 top
SV2  6.35,41.91 270 top
SV3  14.61,40.64 270 top
TP1  21.59,87.63 0 top
TP2  21.59,86.36 0 top
TP3  21.59,85.09 0 top
TP4  21.59,83.82 0 top
TP5  21.59,82.55 0 top
TP6  21.59,81.28 0 top
TP7  21.59,80.01 0 top
TP8  21.59,78.74 0 top
TP9  21.59,77.47 0 top
TP10  21.59,76.2 0 top
TP11  21.59,74.93 0 top
TP12  21.59,73.66 0 top
TP13  21.59,90.17 0 top
TP14  27.94,71.12 0 top
TP15  29.21,71.12 0 top
TP16  30.48,71.12 0 top
TP17  31.75,71.12 0 top
TP18  33.02,71.12 0 top
TP19  34.29,71.12 0 top
TP20  35.56,71.12 0 top
TP21  36.83,71.12 0 top
TP22  38.1,71.12 0 top
TP23  43.18,88.9 0 top
TP24  43.18,87.63 0 top
TP25  43.18,86.36 0 top
TP26  43.18,85.09 0 top
TP27  43.18,83.82 0 top
TP28  43.18,81.28 0 top
TP29  43.18,80.01 0 top
TP30  27.94,24.77 0 top
TP31  27.94,23.5 0 top
TP32  43.18,76.2 0 top
TP33  43.18,74.93 0 top
TP34  43.18,73.66 0 top
TP50  51.44,71.12 0 top
TP53  51.44,54.61 0 top
TP54  60.33,71.75 0 bottom
TP55  51.44,59.69 0 top
TP56  51.44,57.15 0 top
TP57  51.44,55.88 0 top
TP58  43.18,90.17 0 top
TP59  21.59,88.9 0 top
TP62  64.14,55.88 0 top
TP63  64.14,57.15 0 top
TP64  55.24,71.75 0 bottom
TP65  64.14,68.58 0 top
TP66  64.14,69.85 0 top
TP68  74.93,62.87 0 top
TP71  5.08,81.28 0 top
TP78  13.97,29.21 0 top
TP79  27.3,31.75 0 top
TP80  18.41,27.3 0 top
TP81  27.3,30.48 0 top
TP82  18.41,24.77 0 top
TP83  13.97,85.09 90 top
TP84  27.94,26.04 0 top
TP85  18.41,26.04 0 top
TP86  43.18,78.74 0 top
TP87  78.74,81.28 0 top
TP88  43.18,77.47 0 top
TP89  33.66,54.61 0 top
TP90  34.92,54.61 0 top
TP91  36.2,54.61 0 top
TP99  66.67,88.9 0 top
TP100  67.31,89.53 0 top
TP102  64.14,71.12 0 top
TP103  71.75,85.09 0 top
TP104  71.12,85.72 0 top
TP105  71.12,84.45 0 top
TP106  71.75,83.82 0 top
TP107  71.75,86.36 0 top
TP108  46.99,96.52 0 top
TP109  69.85,88.9 0 top
TP110  76.2,90.17 0 top
TP111  77.47,90.81 0 top
TP112  62.87,85.72 0 top
TP113  69.22,89.53 0 top
TP114  63.5,86.36 0 top
TP115  67.94,81.28 0 top
TP116  67.31,80.64 0 top
TP117  66.67,81.28 0 top
TP118  66.04,80.64 0 top
TP119  71.12,83.19 0 top
TP120  69.22,81.28 0 top
TP121  68.58,80.64 0 top
TP122  62.87,84.45 0 top
TP123  63.5,85.09 0 top
TP124  62.87,83.19 0 top
TP125  65.41,81.28 0 top
TP126  63.5,83.82 0 top
U1  67.31,85.09 270 top
U2  10.16,81.28 180 top
U3  22.86,25.4 0 top
U4  CAT24C32WI-GT3  [SOIC127P600X175-8N']  22.86,32.38 0 top
U$2  57.78,62.87 0 top
U$3  24.13,90.17 0 top

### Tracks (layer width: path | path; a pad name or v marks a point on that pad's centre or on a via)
3V3  (via drill 0.35)
  Top 0.152: TP71.TP U2.4 13.02,81.28 | 13.02,81.28 U2.2 | 13.02,81.28 v13.02,82.55 | v17.78,86.36 17.78,88.11 19.21,89.53 20.95,89.53 TP59.TP U$3.2 v27.94,88.9 34.29,88.9 43.97,98.58 50.01,98.58 61.12,87.47 | 73.66,61.44 73.18,60.96 C4.2 69.85,60.96 68.58,59.69 U$2.19 62.39,59.69 61.75,60.33 | 70.64,57.15 R5.1 | 70.64,57.15 R6.1 | U$2.15 62.07,54.61 61.12,55.56 61.12,56.52 | 61.12,56.52 61.12,59.69 61.75,60.33 | 61.75,60.33 62.39,60.96 U$2.20 | 70.64,57.15 66.99,57.15 66.36,56.52 61.12,56.52 | U1.6 66.2,87.47 65.88,87.47 U1.7 65.72,87.47 63.98,87.47 63.5,87.95 61.59,87.95 61.12,87.47 | U$2.28 63.18,71.12 | 63.18,71.12 TP102.TP | 61.12,87.47 v60.33,86.68 59.69,86.04 59.69,82.39 60.8,81.28 | 60.8,81.28 63.18,78.9 63.18,77.79 | 63.18,71.12 63.18,72.23 | 63.18,72.23 63.18,77.79 | 63.18,72.23 61.12,70.17 61.12,68.26 62.07,67.31 U$2.25 68.58,67.31 68.9,67.63 68.9,68.9 69.85,69.85 73.18,69.85 77.15,65.88 77.15,59.85 76.68,59.37 75.72,59.37 73.66,61.44 | 60.8,81.28 v51.75,81.28 | 63.18,77.79 v67.31,77.79 | 73.66,61.44 J1.4
  Bottom 0.152: 29.37,88.9 29.37,89.53 C21.1 29.37,88.9 | 29.37,88.9 29.37,87 C22.1 | 29.37,88.9 v27.94,88.9 | 12.54,83.03 12.06,82.55 C3.1 | 12.54,83.03 13.65,84.14 15.88,84.14 R11.2 16.99,85.09 16.99,85.57 v17.78,86.36 | v13.02,82.55 12.54,83.03 | C20.1 68.74,80.01 68.74,77.47 C19.1 68.58,77.47 68.26,77.79 v67.31,77.79 | R10.1 R12.1 | v60.33,86.68 60.01,86.68 59.05,85.72 R24.1 | v51.75,81.28 R10.1 | R10.1
BAT  (via drill 0.35)
  Top 0.152: TP82.TP U3.3 v21.91,24.77
  Bottom 0.152: R20.2 R19.2 | v21.91,24.77 21.91,22.86 R20.2 | R20.2
CS_IO19  (via drill 0.35)
  Top 0.152: U$3.31 41.27,81.28 TP28.TP v44.45,81.28 | U$2.9 51.91,60.96 50.8,59.85 50.8,59.53 51.28,59.05 54.13,59.05 55.09,60.01 55.09,73.34 v47.31,81.12
  Bottom 0.152: v44.45,81.28 47.31,81.28 | 47.31,81.28 R10.2 | 47.31,81.28 v47.31,81.12
CTS
  Top 0.152: TP106.TP 70.48,83.82 70.33,83.98 69.69,83.98 U1.23
DCD
  Top 0.152: TP109.TP 69.85,88.42 68.9,87.47 U1.1
DSR
  Top 0.152: TP107.TP 70.48,86.36 70.33,86.2 69.69,86.2 U1.27
DTR  (via drill 0.35)
  Top 0.152: v48.1,95.41 TP108.TP | v69.69,87.31 69.69,86.68 U1.28
  Bottom 0.152: v69.69,87.31 61.59,95.41 v48.1,95.41 47.78,95.09 46.99,95.09 Q2.3 46.99,94.93 23.5,94.93 R37.1
EN  (via drill 0.35)
  Top 0.152: U$3.3 TP1.TP 21.11,88.11 20.48,88.11 | 20.48,88.11 20.16,88.11 S2.3 | 20,94.93 20,90.81 17.14,87.95 17.14,86.04 17.46,85.72 18.1,85.72 20,87.63 | 20,94.93 20,97.16 S2.4 | 20.48,88.11 20,87.63 | 20.48,88.11 S2.3 | 20,94.93 v18.89,94.93 | 20,87.63 v20,85.57 | 20,87.63 S2.3
  Bottom 0.152: 18.73,85.57 18.73,87.63 C15.1 | 18.73,85.57 R11.1 18.73,85.57 | 18.57,95.25 19.05,95.73 19.05,96.52 C9.1 | 18.57,95.25 17.78,94.46 Q1.3 | v18.89,94.93 18.57,95.25 | v20,85.57 18.73,85.57
EXT_5V  (via drill 0.35)
  Top 0.152: TP83.TP 13.97,83.98 13.65,83.66 U2.3 13.65,83.5 13.65,82.55 14.45,81.76 14.45,78.42 | 7.14,71.12 14.45,78.42 | 14.45,78.42 v14.76,78.42 | C13.- 18.41,46.99 SV3.1 9.53,38.1 SV2.5 | v31.91,25.08 31.91,25.56 30.16,27.3 U3.8 25.24,27.3 25.24,28.42 23.65,30 23.65,33.02 24.92,34.29 U4.8 25.4,34.29 25.4,37.78 | 18.1,66.36 15.56,66.36 13.81,64.61 | 18.1,66.36 18.41,66.36 MAX232.16 18.1,66.36 | 13.81,64.61 13.34,64.14 C16.+ 13.81,64.61 | 33.34,65.41 31.59,65.41 29.84,63.66 29.53,63.66 | 33.34,65.41 33.66,65.41 IC1.16 | 29.53,63.66 20.8,63.66 18.1,66.36 | 33.34,65.41 v33.34,63.5 | 25.4,37.78 25.4,43.5 30,48.1 30,55.4 29.53,55.88 29.53,63.66 | 25.4,37.78 v20.16,37.78 | 7.14,71.12 13.65,64.61 13.81,64.61 | 7.14,71.12 SV1.2 | 79.06,81.28 82.55,81.28 POWER.3 83.82,78.11 88.9,73.03 88.9,40.32 v86.84,38.26 | 79.06,81.28 TP87.TP | v59.85,90.81 69.53,90.81 79.06,81.28 | 71.75,17.14 71.75,28.42 63.82,36.35 RELAY.A1 | 71.75,17.14 71.75,15.88 PUSH_BUTTON.3 64.77,8.89 41.27,8.89 40.48,9.68 40.48,10.95 v33.81,17.62 | PUSH_BUTTON.7 71.75,17.14
  Bottom 0.152: 19.21,80.01 17.62,78.42 v14.76,78.42 11.91,78.42 11.59,78.74 C1.1 | 19.21,80.01 19.21,82.55 C25.1 | 19.21,80.01 C24.1 | R15.1 R14.1 | 31.91,31.75 31.91,34.29 C17.1 | R17.1 R18.2 | R17.1 31.91,31.75 | 31.91,31.75 C18.1 | R17.1 | R18.2 v31.91,25.08 R15.1 | R15.1 | R18.2 | R35.1 R34.1 | R35.1 R36.1 | R35.1 | R34.1 34.45,63.5 v33.34,63.5 | R34.1 | SV3.1 20,37.78 v20.16,37.78 | v59.85,90.81 D1.K | POWER.3 83.66,80.17 80.8,80.17 80.8,84.93 79.38,86.36 R2.2 | 71.91,31.75 73.5,31.75 77.79,36.04 84.61,36.04 v86.84,38.26 R22.2 | 71.91,31.75 69.85,33.81 66.36,33.81 63.82,36.35 RELAY.A1 | 71.91,31.75 D3.K | R14.1 33.34,17.62 v33.81,17.62 | R14.1
GND  (via drill 0.35)
  Top 0.152: U1.29 67.31,86.52 67.79,87 67.79,87.31 U1.3
  other vias: 62.87,45.72 19.05,60.33 26.04,71.12 51.44,89.53 49.53,60.96 51.44,69.85 57.78,59.69 46.99,66.67 74.3,92.71 22.23,92.08 46.35,59.69 50.8,96.52 26.04,37.47 18.41,64.14 29.84,67.94 64.77,58.42 64.77,60.96 23.5,21.59 69.22,93.34 74.3,78.11 64.14,81.28 71.75,80.64 69.85,82.55 71.12,87.63 42.55,91.44 27.3,84.45 29.84,41.91 45.72,26.04 61.59,20.32 52.7,17.14
  pour Top: 0,100.33 95.25,100.33 95.25,0 0,0
  pour Bottom: 0,100.33 95.25,100.33 95.25,0 0,0
INT_IO23  (via drill 0.35)
  Top 0.152: U$3.37 43.02,88.9 | U$2.4 52.07,67.31 50.48,68.9 v50.48,69.06 | v51.59,79.85 51.59,80.17 45.72,86.04 v45.72,90.49 | 43.02,88.9 v44.45,90.33 | 43.02,88.9 TP23.TP
  Bottom 0.152: v50.48,69.06 50.48,70.96 51.91,72.39 51.91,79.85 v51.59,79.85 | v45.72,90.49 45.56,90.33 v44.45,90.33
IO0  (via drill 0.35)
  Top 0.152: U$3.25 41.27,73.66 TP34.TP 44.13,73.66 45.09,74.61 45.09,86.36 | 45.09,90.01 44.77,89.69 44.77,88.27 S1.4 | 45.09,90.01 45.09,91.44 45.24,91.6 45.24,96.68 44.77,97.16 S1.3 | 45.09,90.01 45.09,86.36 | 45.09,86.36 v44.13,86.36
  Bottom 0.152: C14.1 v44.13,86.36 43.81,86.36 43.81,92.08 44.45,92.71 45.88,92.71 46.04,92.87 Q2.2
IO2  (via drill 0.35)
  Top 0.152: v68.74,26.67 68.74,29.05 57.94,39.85 57.94,43.97 39.37,62.55 v39.37,68.74 | v37.94,70.17 37.94,70.96 TP22.TP 38.1,72.55 38.26,72.71 U$3.24 38.42,72.87 38.42,77.15 39.37,78.11 39.37,91.6 40.32,92.55 43.97,92.55 v44.61,91.92 | v46.04,91.44 53.82,91.44 56.83,88.42 57.15,88.42 S3.2
  Bottom 0.152: v68.74,26.67 68.74,25.88 Q4.1 | v37.94,70.17 v39.37,68.74 | v46.04,91.44 45.56,91.92 v44.61,91.92
IO4  (via drill 0.35)
  Top 0.152: U$3.26 41.27,74.93 TP33.TP v43.81,74.3
  Bottom 0.152: v43.81,74.3 42.86,73.34 42.86,54.29 13.97,54.29 8.1,48.42 6.51,48.42 SV2.1
IO12  (via drill 0.35)
  Top 0.152: 23.5,73.66 TP12.TP | v47.94,84.77 51.44,88.27 54.61,88.27 S3.1 | 23.5,73.66 v24.61,72.55 | 23.5,73.66 U$3.14
  Bottom 0.152: v47.94,84.77 46.67,83.5 35.56,83.5 v24.61,72.55
IO13  (via drill 0.35)
  Top 0.152: U$3.16 28.1,72.71 27.94,72.55 TP14.TP v25.4,68.58
  Bottom 0.152: v25.4,68.58 25.24,68.74 13.18,68.74 8.1,63.66 6.51,63.66 SV1.5
IO15  (via drill 0.35)
  Top 0.152: U$3.23 36.99,72.71 36.83,72.55 TP21.TP 36.35,71.12 v29.53,64.29 | v27.3,62.71 14.45,62.71 13.81,62.07 7.46,62.07 SV1.6
  Bottom 0.152: v29.53,64.29 27.94,62.71 v27.3,62.71
IO16  (via drill 0.35)
  Top 0.152: U$3.27 41.27,76.2 TP32.TP v43.81,75.56 | v28.89,62.07 28.89,60.01 v27.94,59.05
  Bottom 0.152: v43.81,75.56 39.05,70.8 37.62,70.8 v28.89,62.07 | SV2.3 3.81,45.72 3.81,53.98 4.45,54.61 8.26,54.61 12.7,59.05 v27.94,59.05
IO32
  Top 0.152: U$3.8 TP6.TP 18.57,81.28 14.13,85.72 8.57,85.72 4.45,81.6 4.45,70.48 SV1.3
IO33  (via drill 0.35)
  Top 0.152: U$3.9 TP7.TP v10.48,68.9
  Bottom 0.152: v10.48,68.9 7.62,66.04 SV1.4
IO34  (via drill 0.35)
  Top 0.152: U$3.6 TP4.TP 16.51,83.82 14.29,86.04 8.41,86.04 4.13,81.76 4.13,13.81 10.64,7.3 v70.33,7.3
  Bottom 0.152: 71.44,6.35 R29.1 71.44,6.35 | 71.44,6.35 73.66,6.35 C23.2 | v70.33,7.3 71.28,6.35 71.44,6.35
IO35  (via drill 0.35)
  Top 0.152: TP5.TP U$3.7 25.88,82.55 29.05,79.38 v38.73,79.38 | v45.09,73.66 45.09,63.82 50.8,58.1 50.8,55.72 51.28,55.24 60.17,55.24 73.18,42.23 v87.95,42.23
  Bottom 0.152: Q6.3 87.95,43.18 v87.95,42.23 87.95,40.8 88.74,40.8 89.69,39.85 89.69,39.37 R22.1 | v38.73,79.38 41.91,76.2 44.13,76.2 45.09,75.25 v45.09,73.66
LEDA
  Top 0.152: U$2.27 TP66.TP 66.52,69.85 68.42,71.75 86.04,71.75 88.58,69.22 88.58,56.83 87.47,55.72 J1.9
LEDB
  Top 0.152: U$2.26 TP65.TP 65.72,68.58 68.58,71.44 84.77,71.44 87.31,68.9 J1.12
N$1  (via drill 0.35)
  Top 0.152: v81.44,84.77 81.44,85.72 LED1.A
  Bottom 0.152: v81.44,84.77 81.44,86.36 R2.1
N$2
  Bottom 0.152: Q1.1 18.57,92.23 16.99,90.65 16.99,90.17 R37.2
N$3
  Bottom 0.152: Q2.1 47.78,92.87 47.78,90.33 47.15,90.33 46.2,89.38 46.2,88.9 R21.2
N$4  (via drill 0.35)
  Top 0.152: U1.8 64.93,86.52 64.45,86.52 64.29,86.36 TP114.TP 63.5,87 v63.18,87.31
  Bottom 0.152: R1.1 62.23,88.27 v63.18,87.31 63.18,84.61 R26.2
N$5
  Bottom 0.152: SV2.4 6.51,40.8 14.45,40.8 SV3.2
N$6  (via drill 0.35)
  Top 0.152: U1.11 TP123.TP 62.71,85.09 62.23,84.61 62.23,81.76 v62.55,81.44
  Bottom 0.152: v62.55,81.44 61.75,80.64 R23.1
N$7
  Bottom 0.152: R8.2 86.04,66.2 87.31,66.2 J1.11
N$8
  Top 0.152: R3.1 70.64,68.58 C2.2 | J1.5 TP68.TP 74.61,62.87 | R4.1 72.87,63.5 73.5,62.87 74.61,62.87 | R3.1 72.87,66.04 73.82,65.09 74.14,65.09 74.61,64.61 74.61,62.87 | R3.1
N$9
  Bottom 0.152: R9.2 86.04,58.26 87.31,58.26 J1.10
N$10
  Top 0.152: TP115.TP 67.94,82.55 67.79,82.71 U1.19
N$11
  Top 0.152: U1.18 TP116.TP
N$12
  Top 0.152: MAX232.1 18.41,56.67 16.67,56.67 13.34,53.34 C10.+
N$13
  Top 0.152: TP117.TP 66.67,82.55 66.83,82.71 U1.17
N$14
  Top 0.152: MAX232.3 20.95,53.34 18.89,51.28 14.92,51.28 13.34,49.69 C10.-
N$15
  Top 0.152: C11.- MAX232.5
N$16  (via drill 0.35)
  Top 0.152: U1.9 64.93,86.04 64.45,86.04 64.14,85.72 TP112.TP v60.33,85.72
  Bottom 0.152: R24.2 v60.33,85.72
N$17
  Top 0.152: TP118.TP 66.04,81.92 66.2,82.07 66.2,82.71 U1.16
N$18
  Top 0.152: MAX232.4 22.23,50.96 23.5,49.69 C11.+
N$19
  Top 0.152: MAX232.6 24.77,55.72 27.15,53.34 28.57,53.34 C12.-
N$20
  Top 0.152: MAX232.2 19.68,54.61 18.41,53.34 C13.+
N$21
  Top 0.152: RELAY_CONN.5 81.76,36.35 76.04,36.35 RELAY.NC
N$22  (via drill 0.35)
  Top 0.152: v69.53,33.18 79.85,33.18 RELAY_CONN.3
  Bottom 0.152: v69.53,33.18 64.45,33.18 RELAY.COM
N$23
  Top 0.152: LED5.K 35.08,50.01 R31.1 LED2.C
  Bottom 0.152: LED5.K 34.13,49.53 R31.1
N$24
  Top 0.152: IC1.13 37.47,65.09 34.45,62.07 30.48,62.07 R40NC.2
N$25
  Top 0.152: TP119.TP 70.01,83.19 69.69,83.5 U1.22
N$26
  Top 0.152: RELAY_CONN.1 83.5,24.45 76.04,24.45 RELAY.NO
N$27
  Bottom 0.152: 69.69,30.48 70.8,30.48 70.8,26.67 Q4.3 | 69.69,30.48 68.42,31.75 D3.A | 69.69,30.48 63.82,24.61 RELAY.A2
N$28  (via drill 0.35)
  Top 0.152: v24.45,28.26 20.95,28.26 18.89,30.32 D2.A
  Bottom 0.152: v24.45,28.26 25.4,29.21 R17.2
N$29  (via drill 0.35)
  Top 0.152: D2.K 15.88,34.29 13.97,32.38 TP78.TP 13.97,26.83 v17.46,23.34 20.8,20 29.37,20 41.12,31.75 BT1.+
  Bottom 0.152: v17.46,23.34 18.41,23.34 R20.1
N$30
  Top 0.152: TP120.TP 69.22,82.39 68.9,82.71 U1.21
N$31
  Top 0.152: TP121.TP 68.58,81.92 68.42,82.07 68.42,82.71 U1.20
N$32
  Bottom 0.152: R27.1 89.53,45.72 89.53,44.13 89.85,44.13 Q6.1
N$33
  Bottom 0.152: PUSH_BUTTON.5 69.69,8.73 69.69,6.35 | 69.69,6.35 69.69,5.08 70.64,4.13 R29.2 70.8,4.13 R28.2 | 67.47,4.13 69.69,6.35
N$34
  Top 0.152: TP122.TP 64.77,84.45 64.93,84.61 U1.12
N$35
  Bottom 0.152: DRY_CONTACT.3 88.27,45.72 R27.2
N$36
  Top 0.152: LED2.A 33.66,51.59 35.08,51.59 LED5.A 37.47,53.98 IC1.4
N$37
  Top 0.152: 38.73,51.59 40.16,51.59 LED6.A | 38.73,51.59 IC1.5 | 38.73,51.59 LED3.A
N$38
  Top 0.152: 43.81,51.59 45.24,51.59 LED7.A | IC1.6 40.01,55.4 43.81,51.59 | 43.81,51.59 LED4.A
N$39
  Top 0.152: TP124.TP 64.61,83.19 64.93,83.5 U1.14
N$40
  Bottom 0.152: PUSH_BUTTON.1 62.39,11.43 62.39,6.19 64.77,3.81 R30.2
N$41
  Top 0.152: TP125.TP 65.41,82.39 65.72,82.71 U1.15
N$42
  Top 0.152: TP126.TP 64.14,83.82 64.29,83.98 64.93,83.98 U1.13
N$45  (via drill 0.35)
  Top 0.152: TP89.TP IC1.1 33.66,56.52 31.91,58.26 | R40NC.1 30.48,59.69 31.91,58.26 | 31.91,58.26 v33.34,59.69
  Bottom 0.152: v33.34,59.69 34.45,59.69 R34.2
N$46  (via drill 0.35)
  Top 0.152: TP90.TP IC1.2 34.92,56.99 v36.83,58.9
  Bottom 0.152: v36.83,58.9 R35.2
N$47  (via drill 0.35)
  Top 0.152: TP91.TP IC1.3 36.2,56.83 37.15,57.78 37.31,57.78 v39.69,60.17
  Bottom 0.152: v39.69,60.17 R36.2
N$48
  Top 0.152: LED6.K 40.16,50.01 R32.1 LED3.C
  Bottom 0.152: LED6.K 39.21,49.53 R32.1
N$49
  Top 0.152: LED7.K 45.24,50.01 R33.1 LED4.C
  Bottom 0.152: LED7.K 44.29,49.53 R33.1
N$67
  Top 0.152: TP20.TP 35.56,72.55 35.72,72.71 U$3.22
N$68
  Top 0.152: TP19.TP 34.29,72.55 34.45,72.71 U$3.21
N$69
  Top 0.152: TP18.TP 33.02,72.55 33.18,72.71 U$3.20
N$70
  Top 0.152: TP17.TP 31.75,72.55 31.91,72.71 U$3.19
N$71
  Top 0.152: TP16.TP 30.48,72.55 30.64,72.71 U$3.18
N$72
  Top 0.152: TP15.TP 29.21,72.55 29.37,72.71 U$3.17
OS1
  Top 0.152: U3.1 TP80.TP 15.88,27.3 Q5.1
OS2
  Top 0.152: U3.2 TP85.TP 15.88,26.04 Q5.2
OSC1
  Top 0.152: U$2.23 62.07,64.77 60.17,66.67 60.17,74.77 Q3.2
  Bottom 0.152: C7.1 TP54.TP Q3.2
OSC2
  Top 0.152: U$2.24 62.87,66.04 63.82,65.09 63.82,64.45 63.5,64.14 61.44,64.14 55.4,70.17 55.4,74.77 Q3.1
  Bottom 0.152: C8.1 TP64.TP Q3.1
RBIAS
  Top 0.152: U$2.14 TP53.TP 50.96,55.09 R13.2
RESET  (via drill 0.35)
  Top 0.152: TP55.TP U$2.10 53.5,59.69 54.77,60.96 54.77,71.6 49.05,77.31 v48.74,77.31
  Bottom 0.152: v48.74,77.31 48.74,78.74 R12.2
RI
  Top 0.152: TP113.TP 69.22,88.9 68.42,88.11 68.42,87.47 U1.2
RTS  (via drill 0.35)
  Top 0.152: U1.24 69.69,84.61 69.85,84.45 TP105.TP 71.91,84.45 72.39,83.98 v72.39,83.19 | v16.99,93.34 16.99,96.36 19.53,98.9 50.48,98.9 54.61,94.77 v54.77,94.77
  Bottom 0.152: v16.99,93.34 16.99,92.39 Q1.2 | R21.1 48.9,88.9 v54.77,94.77 60.96,94.77 63.66,92.08 64.45,92.08 64.45,91.12 v72.39,83.19
RX_232
  Top 0.152: MAX232.7 26.04,57.63 25.4,58.26 13.49,58.26 7.14,51.91 5.24,51.91 4.45,51.12 4.45,24.77 | RS232.3 4.45,24.77 | J2.3 13.34,11.43 10.79,8.89 9.53,8.89 4.45,13.97 4.45,24.77
RX_S  (via drill 0.35)
  Top 0.152: v20.95,68.1 MAX232.14 | v39.37,57.94 42.7,57.94 57.63,43.02 57.63,32.54 57.78,32.38 57.78,17.14 SCANNER.7
  Bottom 0.152: v20.95,68.1 31.11,57.94 v39.37,57.94
RX_UART1_IO14
  Top 0.152: TP11.TP U$3.13 24.77,74.93 25.4,74.3 25.4,72.39 23.5,70.48 MAX232.12
RX_UART2_IO25
  Top 0.152: U$3.10 TP8.TP
RXD
  Top 0.152: U1.25 TP103.TP 72.71,84.14 72.71,83.98 74.14,82.55 R39.2
RXD0  (via drill 0.35)
  Top 0.152: U$3.34 TP26.TP 44.45,83.82 v44.45,82.87 | R39.1 71.28,82.55 68.74,80.01 v63.02,80.01
  Bottom 0.152: v63.02,80.01 62.23,79.22 54.77,79.22 51.12,82.87 v44.45,82.87
SCK_IO21  (via drill 0.35)
  Top 0.152: U$3.33 42.7,83.82 | 42.7,83.82 TP27.TP | U$2.8 53.5,62.23 54.45,63.18 54.45,71.44 49.21,76.68 48.1,76.68 v45.72,79.06 | 42.7,83.82 v42.7,82.07
  Bottom 0.152: v42.7,82.07 v45.72,79.06
SCL_IO5  (via drill 0.35)
  Top 0.152: U3.6 TP30.TP 28.26,24.45 v29.05,24.45 | v25.88,28.26 23.97,30.16 23.97,30.8 24.92,31.75 U4.6 TP79.TP 27.3,44.93 30.32,47.94 30.32,55.56 29.84,56.04 29.84,62.55 30.16,62.87 33.97,62.87 36.2,65.09 IC1.14 36.2,67.47 39.53,70.8 39.53,77.79 40.32,78.58 41.12,78.58 U$3.29 41.27,78.74 TP86.TP
  Bottom 0.152: R15.2 v29.05,24.45 27.62,24.45 27.62,26.51 v25.88,28.26
SDA_IO17  (via drill 0.35)
  Top 0.152: U4.5 TP81.TP | U3.5 26.19,23.5 | 26.19,23.5 TP31.TP | 26.19,23.5 28.73,20.95 | 28.73,20.95 v29.05,20.64 | TP81.TP 30.16,27.62 30.32,27.62 32.54,25.4 32.54,24.77 28.73,20.95 | TP88.TP 41.27,77.47 U$3.28 41.12,77.31 40.32,77.31 39.85,76.83 39.85,70.64 38.1,68.9 | IC1.15 34.92,66.52 v35.56,67.15 | v36.83,67.15 36.83,67.63 38.1,68.9 | TP81.TP 27.3,30.96 33.02,36.67 33.02,53.18 34.29,54.45 34.29,60.64 38.1,64.45 38.1,68.9
  Bottom 0.152: v29.05,20.64 R14.2 | v36.83,67.15 v35.56,67.15
SENSOR_VN
  Top 0.152: U$3.5 TP3.TP
SENSOR_VP
  Top 0.152: TP2.TP 24.13,86.36 U$3.4
SI_IO18  (via drill 0.35)
  Top 0.152: U$3.30 41.27,80.01 TP29.TP 44.45,78.74 v44.45,77.15 | U$2.7 50.01,63.5 49.85,63.34 47.94,63.34 45.72,65.56 v45.72,75.88
  Bottom 0.152: v44.45,77.15 v45.72,75.88
SO_IO22  (via drill 0.35)
  Top 0.152: TP24.TP U$3.36 40.48,87.63 39.85,88.27 39.85,90.81 40.32,91.28 v40.64,91.28 | U$2.6 51.44,64.77 49.37,66.83 48.1,66.83 46.35,68.58 46.35,76.2 v45.72,76.83 | v38.73,89.38 v38.73,82.87
  Bottom 0.152: v45.72,76.83 39.69,82.87 v38.73,82.87 | v40.64,91.28 v38.73,89.38
SQ  (via drill 0.35)
  Top 0.152: U3.7 TP84.TP v30.48,26.04
  Bottom 0.152: v30.48,26.04 29.84,26.04 29.21,26.67 R18.1
TPIN+
  Top 0.152: J1.3 74.59,61.93 74.59,61.97 74.04,62.52 71.68,62.52 71.53,62.37 69.74,62.37 69.25,62.87 68.58,62.87 | 68.58,62.87 64.71,62.87 63.57,61.72 61.09,61.72 55.24,55.88 U$2.13 TP57.TP | R4.2 67.94,63.5 68.58,62.87
TPIN-
  Top 0.152: J1.6 72.88,64.91 69.74,64.91 69.25,65.41 67.79,65.41 | 67.79,65.41 66.04,65.41 63.5,62.87 59.69,62.87 53.98,57.15 U$2.12 TP56.TP | 67.79,65.41 R3.2
TPOUT+
  Top 0.152: U$2.17 TP63.TP 66.52,57.15 R5.2 69.06,59.69 72.39,59.69 73.03,60.33 74.3,60.33 76.2,58.42 J1.1
TPOUT-
  Top 0.152: U$2.16 TP62.TP R6.2 69.7,53.98 71.75,53.98 73.66,55.88 J1.2
TX_232
  Top 0.152: MAX232.8 27.3,56.67 27.62,56.67 29.69,54.61 29.69,48.26 17.14,35.72 15.08,35.72 8.26,28.89 8.26,22.23 RS232.4 10.16,16.51 J2.1
TX_S  (via drill 0.35)
  Top 0.152: MAX232.13 22.23,67.79 21.27,68.74 20.64,68.74 v20,68.1 | v30.48,57.63 30.48,55.88 32.38,53.98 v32.38,37.94 | v40.32,30 40.32,18.1 SCANNER.5
  Bottom 0.152: v30.48,57.63 v20,68.1 | v40.32,30 v32.38,37.94
TX_UART1_IO27
  Top 0.152: TP10.TP U$3.12 24.77,76.2 25.72,75.25 25.72,72.23 24.77,71.28 MAX232.11
TX_UART2_IO26
  Top 0.152: U$3.11 TP9.TP 20.95,76.83 20.95,73.5 22.86,71.6 22.86,65.41 23.02,65.25 25.24,65.25 26.04,66.04 MAX232.10
TXD
  Top 0.152: U1.26 69.69,85.57 69.85,85.72 TP104.TP 73.5,85.72 74.14,85.09 R38.2
TXD0  (via drill 0.35)
  Top 0.152: U$3.35 42.86,86.36 | 42.86,86.36 TP25.TP | v63.82,79.38 72.07,79.38 74.77,82.07 74.77,83.03 73.18,84.61 73.18,85.09 R38.1 | v62.55,78.58 51.28,78.58 v45.72,84.14 | 42.86,86.36 v44.45,84.77
  Bottom 0.152: v63.82,79.38 63.02,78.58 v62.55,78.58 | v45.72,84.14 45.09,84.77 v44.45,84.77
USB_DN
  Top 0.152: TP111.TP 77.47,92.08 J4.2 77.47,92.23 77.47,93.19 76.83,93.82 76.83,96.04 75.88,97 66.99,97 65.88,95.89 | U1.5 66.83,87.47 66.67,87.63 TP99.TP 60.8,88.9 59.21,90.49 59.21,92.55 63.34,96.68 65.09,96.68 65.88,95.89 | 65.88,95.89 65.88,95.09 J3.2
USB_DP  (via drill 0.35)
  Top 0.152: U1.4 TP100.TP v67.94,90.17 | 76.2,90.96 TP110.TP | 76.2,90.96 76.83,91.6 J4.3 | J3.3 66.67,95.73 67.63,96.68 70.01,96.68 71.6,95.09 71.6,93.98 71.75,93.82 | 71.75,93.82 74.61,90.96 76.2,90.96 | 71.75,93.82 v70.48,92.55
  Bottom 0.152: v67.94,90.17 70.33,92.55 v70.48,92.55
VBUS  (via drill 0.35)
  Top 0.152: 65.25,92.87 65.25,94.93 J3.1 | 65.25,92.87 65.25,92.55 66.04,91.76 69.85,91.76 72.07,89.53 76.99,89.53 78.11,90.65 78.11,92.08 J4.1 | 65.25,92.87 v63.82,91.44
  Bottom 0.152: R1.2 59.69,88.27 62.23,90.81 D1.A 63.02,91.44 v63.82,91.44
VCAP
  Top 0.152: U$2.1 TP50.TP 50.96,71.12 48.9,69.06 C6.+

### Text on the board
tNames: +5V | GND | LCD | SIG | GND | TX | RX | NC | GND | GND | NC | TX | -VE | +VE | PB | PB | PRINTER | RX
bNames: NC | COM | NO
